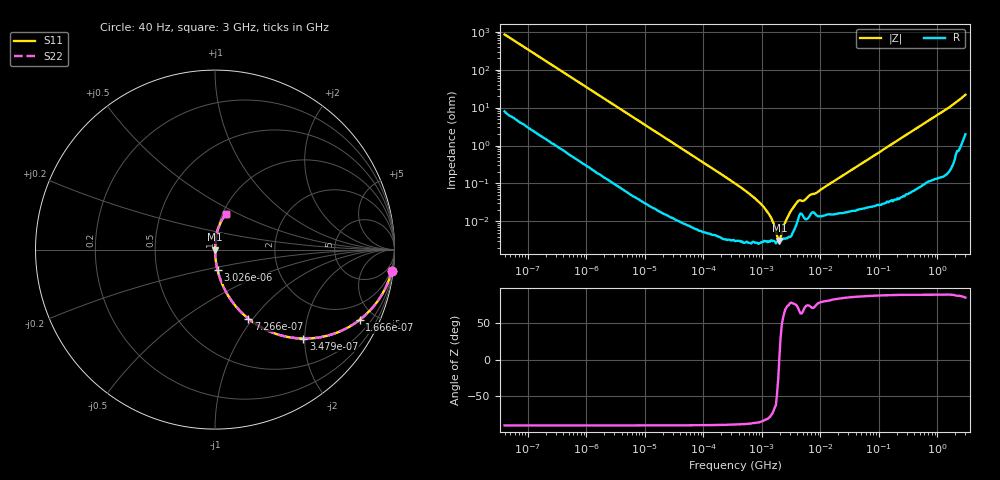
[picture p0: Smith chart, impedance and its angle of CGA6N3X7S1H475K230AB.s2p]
! S-parameter Generated by TDK Corporation
! Copyright(C) 2015 TDK Corporation.
! All Rights Reserved.
! TDK P/N: CGA6N3X7S1H475K230AB (Multilayer Ceramic Chip Capacitors)
! Property: C=4.7uF
! Size(LxWxT): 3.2x2.5x2.3mm, 0.126x0.098x0.091inches
! Model Type: s2p (Touchstone File Format Version 1.0)
! Frequency: DC=Yes Start=0.00004MHz Stop=3000MHz 396points Log-sweep
! Note: This model was converted from impedance.
! Model Generated on Jun. 23, 2015
! Hash(MD5):
! Port Assignments:
!  1 ---| |--- 2
! Applicable Conditions:
!  Temperature = 25 degC
!  DC Bias Voltage = 0 V
!  Small Signal Operation
! Terms and conditions regarding TDK Simulation Models
! (1)This simulation model is being provided solely for informational purposes. Please refer to the specifications of the products in terms of detailed characteristics of such products.
! (2)In no event shall TDK Corporation of any of its subsidiaries be liable for any loss or damage arising, directly or indirectly,
!  From any information contained in this simulation model, including, but not limited to loss or damages arising from any inaccuracies, omissions or errors in connection with such information.
! (3)Any and all copyrights on this simulation model are owned by TDK Corporation.
!  Duplication or redistribution of this simulation model without prior written permission from TDK Corporation is prohibited.
! (4)This simulation model is subject to any modification or change without any prior notice.
! (5)Neither TDK Corporation nor any of its subsidiaries shall make any warranty, express or implied,
!  Including but not limited to the correctness, implied warranties of merchantability and fitness for a particular purpose with respect to this simulation models.
! (6)The use of this simulation model shall be deemed to have consented to the terms and conditions hereof.
# MHz S MA R 50
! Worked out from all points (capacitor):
!   395 points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, 40 Hz to 3 GHz, reference 50 ohm
!   read as one part in series: C = 4.69 uF near 41.88 Hz
!   lowest |Z| = 3.12 mohm at 1.991 MHz (marker M1)
!   series resonance near 1.977 MHz, so ESL is about 1.4 nH
!   S11 on the Smith chart (normalised r, x): 40 Hz: 1, -17; 166.6 Hz: 1.04, -4.10; 347.9 Hz: 1.02, -1.97; 726.6 Hz: 1.01, -0.95; 3.026 kHz: 1.00, -0.23; 3 GHz: 1.04, +0.43
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4e-05  0.992 -6.7  0.1174 82.7  0.1174 82.7  0.992 -6.7
9.158711e-05  0.9635 -15.0  0.2592 74.5  0.2592 74.5  0.9635 -15.0
0.0001665986  0.8958 -25.9  0.4368 63.6  0.4368 63.6  0.8958 -25.9
0.0003479132  0.6991 -45.1  0.709 44.4  0.709 44.4  0.6991 -45.1
0.000726558  0.4272 -64.2  0.9005 25.3  0.9005 25.3  0.4272 -64.2
0.000834128  0.381 -67.1  0.9214 22.4  0.9214 22.4  0.381 -67.1
0.003026089  0.1143 -83.0  0.9925 6.6  0.9925 6.6  0.1143 -83.0
0.01739424  0.02024 -88.3  0.9996 1.2  0.9996 1.2  0.02024 -88.3
0.3464102  0.001004 -88.2  1 0.1  1 0.1  0.001004 -88.2
0.9534872  0.0002928 -84.6  1 0.0  1 0.0  0.0002928 -84.6
1.315913  0.000156 -78.8  1 0.0  1 0.0  0.000156 -78.8
1.510739  0.0001044 -73.2  1 0.0  1 0.0  0.0001044 -73.2
1.991197  3.121e-05 4.9  1 -0.0  1 -0.0  3.121e-05 4.9
2.506407  9.535e-05 68.5  1 -0.0  1 -0.0  9.535e-05 68.5
3.013016  0.0001732 77.1  1 -0.0  1 -0.0  0.0001732 77.1
4.15828  0.0003437 70.3  0.9999 -0.0  0.9999 -0.0  0.0003437 70.3
5.234209  0.0003541 69.2  0.9999 -0.0  0.9999 -0.0  0.0003541 69.2
7.22376  0.000524 70.6  0.9998 -0.0  0.9998 -0.0  0.000524 70.6
8.293268  0.0005502 73.9  0.9998 -0.0  0.9998 -0.0  0.0005502 73.9
150.6385  0.009904 87.5  0.9996 -0.6  0.9996 -0.6  0.009904 87.5
1040.901  0.06582 85.0  0.9964 -3.8  0.9964 -3.8  0.06582 85.0
3000  0.209 72.8  0.9591 -12.0  0.9591 -12.0  0.209 72.8
